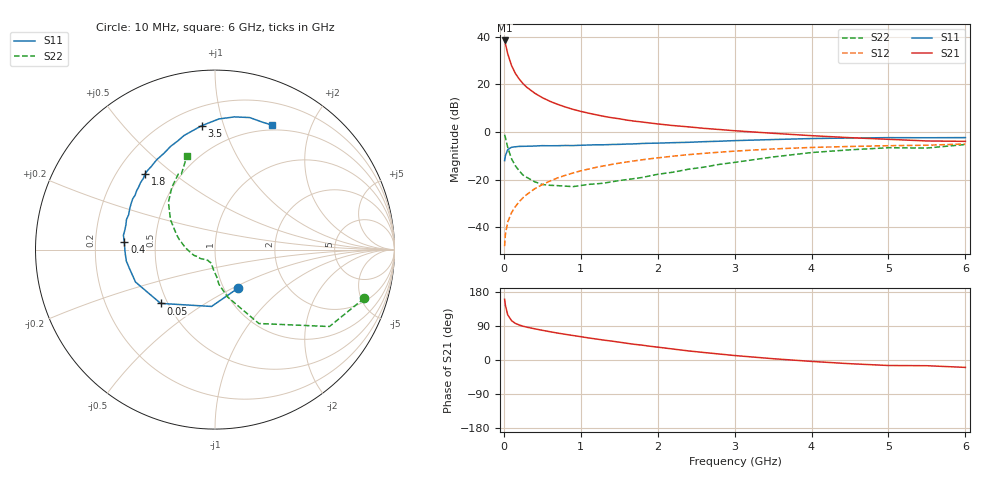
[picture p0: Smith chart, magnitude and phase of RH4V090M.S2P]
! SIEMENS Small Signal Semiconductors
! BFR106
! Si NPN RF Bipolar Junction Transistor in SOT23
! VCE = 4 V  IC = 90 mA
! Common Emitter S-Parameters:  August  1996
# GHz  S  MA  R  50
!  f  S11  S21  S12  S22
! GHz  MAG  ANG  MAG  ANG  MAG  ANG  MAG  ANG
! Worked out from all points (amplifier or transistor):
!   36 points, 10 MHz to 6 GHz, reference 50 ohm
!   highest |S21| = 38.4 dB at 10 MHz (marker M1)
!   |S21| within 3 dB of that: start of sweep to 32.22 MHz
!   unconditionally stable (mu >= 1): 182.2 MHz to 2.447 GHz; 5.479 GHz to 5.577 GHz
!   at 250 MHz: K = 1.05, MAG = 22.6 dB, |S12| = -27.6 dB
!   at 1.4 GHz: K = 1.06, MAG = 8.3 dB, |S12| = -13.6 dB
!   at 6 GHz: K = 1.00, MSG = 0.6 dB, |S12| = -5.0 dB
!   S11 on the Smith chart (normalised r, x): 10 MHz: 1.17, -0.53; 50 MHz: 0.46, -0.34; 400 MHz: 0.33, +0.04; 1.8 GHz: 0.32, +0.40; 3.5 GHz: 0.32, +0.85; 6 GHz: 0.44, +1.46
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0.01  0.2502 -58.5  83.64 160.2  0.004 76.6  0.874 -18.1
0.02  0.3173 -93.5  72.36 144.8  0.007 72.1  0.7684 -33.9
0.05  0.4262 -135.3  44.23 119.4  0.0128 62.1  0.4789 -59.3
0.1  0.4783 -157.8  24.89 103.9  0.0202 65.4  0.2736 -75.1
0.15  0.4887 -167.9  16.98 96.6  0.0271 68.8  0.1949 -83.5
0.2  0.4982 -172.6  12.93 92.4  0.0344 71.7  0.1524 -86.4
0.25  0.5001 -176.9  10.34 89.1  0.0418 72.9  0.1243 -91.4
0.3  0.5022 -179.9  8.66 86.6  0.0489 73.7  0.111 -94.7
0.4  0.5067 175.4  6.561 82.4  0.064 73.9  0.0901 -100.7
0.5  0.5165 171.1  5.261 78.4  0.0786 73.6  0.079 -105.2
0.6  0.5139 167.8  4.405 74.6  0.0935 72.7  0.0759 -109.2
0.7  0.5153 164.5  3.805 71.0  0.1087 71.8  0.0747 -115.0
0.9  0.5189 157.9  2.985 64.6  0.138 69.2  0.0713 -123.9
1.1  0.5325 151.6  2.488 58.3  0.1665 66.4  0.0794 -132.6
1.4  0.5462 143.0  1.997 49.9  0.2081 61.9  0.0898 -144.7
1.8  0.5745 132.7  1.617 39.1  0.2609 55.5  0.111 -160.9
2.2  0.5968 123.0  1.365 28.9  0.311 49.3  0.1432 -176.0
2.8  0.6396 109.0  1.128 15.8  0.376 39.7  0.2087 163.8
3.5  0.6941 96.2  0.939 3.4  0.4405 29.0  0.299 146.1
4.5  0.7472 81.7  0.76 -9.8  0.4967 14.4  0.4223 124.7
5.5  0.7577 69.5  0.648 -15.1  0.5271 5.1  0.4599 114.1
6  0.7625 65.6  0.636 -19.5  0.5601 -1.9  0.5465 106.5
